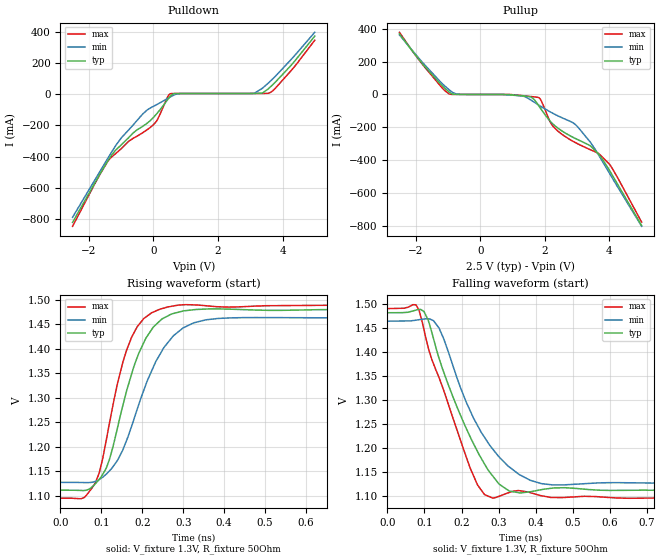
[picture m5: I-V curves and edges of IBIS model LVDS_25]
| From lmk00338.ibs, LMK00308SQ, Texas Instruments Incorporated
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|   Model LVDS_25
[Model]   LVDS_25
Model_type   Output
Polarity   Non-Inverting
Rref =   50.0000
Vref =   1.3
Vmeas =   1.3
|   typ   min   max
|   Nom   Weak   Strong
C_comp   0.6362pF   0.6362pF   0.8920pF
|Output in low   Nom   Weak   Strong
|C_Comp   0.6362pF   0.6362pF   0.8920pF
|Output in High   Nom   Strong   Weak
|C_Comp   1.1227pF   1.0238pF   1.1227pF
[Voltage Range]   2.5   2.375   2.625
[Temperature Range]   45   125   -40
[Pullup Reference]   2.5   2.375   2.625
[Pulldown Reference]   -0   -0   0
[Power Clamp Reference]   2.5   2.375   2.625
[GND Clamp Reference]   0   0   -0
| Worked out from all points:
|   slope of the pulldown table from 0 to 0.375 V, typ, clamps not added: 3.94 ohm
|   slope of the pullup table from 0 to 0.375 V, typ, clamps not added: 13.5 kohm
|   falling waveform, V_fixture 1.3V, R_fixture 50Ohm: 20-80 % time 117ps typ, 122ps min, 107ps max; typ from 1.48 V to 1.11 V
|   rising waveform, V_fixture 1.3V, R_fixture 50Ohm: 20-80 % time 77ps typ, 95.9ps min, 65.1ps max; typ from 1.11 V to 1.48 V
[Pulldown]
|   Voltage   I(typ)   I(min)   I(max)
-2.5V     -821.5mA   -788.4mA   -846.4mA
-1.413V   -428.8mA   -411.9mA   -430.6mA
-992.5mV  -325.1mA   -280.3mA   -349.4mA
-310mV    -203.6mA   -123.8mA   -244.5mA
68.75mV   -134.1mA   -70.9mA    -181.1mA
522.5mV   -14.65mA   -18.34mA   2.238mA
845mV     3.865mA    3.299mA    4.13mA
3.125V    3.984mA    6.314mA    4.216mA
3.365V    6.9mA      36.07mA    4.277mA
3.56V     34.32mA    71.04mA    5.348mA
4.25V     181.4mA    218.6mA    147.2mA
4.996V    371.6mA    396mA      345.1mA
[Pullup]
|   Voltage   I(typ)   I(min)   I(max)
-2.5V     369.5mA    363.6mA    379.4mA
-1.75V    178.3mA    187.4mA    174.3mA
-951.3mV  12.8mA     26.8mA     2.027mA
-748.8mV  390.5uA    2.963mA    222.6uA
1.494V    -12.18mA   -24.91mA   -11.05mA
1.809V    -68.01mA   -64.69mA   -19.09mA
2.27V     -184.1mA   -117.2mA   -197.8mA
2.945V    -268.7mA   -183.6mA   -293.7mA
3.414V    -314.4mA   -292.8mA   -337.7mA
3.654V    -362.6mA   -365.9mA   -358.9mA
4.003V    -463.9mA   -481.3mA   -426.2mA
4.996V    -800.5mA   -804.6mA   -779.2mA
[Ramp]
R_load = 50
|   typ   min   max
dV/dt_r   0.221608/7.69985e-11   0.20221/9.59504e-11   0.236444/6.51342e-11
dV/dt_f   0.221966/1.16694e-10   0.20221/1.22128e-10   0.23693/1.06747e-10
[Falling Waveform]
V_fixture = 1.3V
V_fixture_min = 1.3V
V_fixture_max = 1.3V
R_fixture = 50Ohm
C_fixture = 0F
|   Time   V(typ)   V(min)   V(max)
0s        1.482V     1.464V     1.49V
77.26ps   1.487V     1.466V     1.498V
98.56ps   1.484V     1.468V     1.447V
139.1ps   1.388V     1.45V      1.347V
223.1ps   1.224V     1.278V     1.159V
262.2ps   1.167V     1.222V     1.104V
284.3ps   1.142V     1.198V     1.096V
329.1ps   1.111V     1.161V     1.108V
445.5ps   1.117V     1.124V     1.098V
1.4ns     1.112V     1.127V     1.095V
[Rising Waveform]
V_fixture = 1.3V
V_fixture_min = 1.3V
V_fixture_max = 1.3V
R_fixture = 50Ohm
C_fixture = 0F
|   Time   V(typ)   V(min)   V(max)
0s        1.111V     1.127V     1.095V
63.19ps   1.111V     1.127V     1.1V
94.69ps   1.133V     1.133V     1.146V
109.5ps   1.152V     1.142V     1.202V
139.8ps   1.24V      1.173V     1.33V
173.6ps   1.347V     1.241V     1.423V
243.1ps   1.457V     1.388V     1.48V
299.7ps   1.477V     1.442V     1.489V
385.5ps   1.481V     1.461V     1.485V
1.4ns     1.48V      1.464V     1.489V
